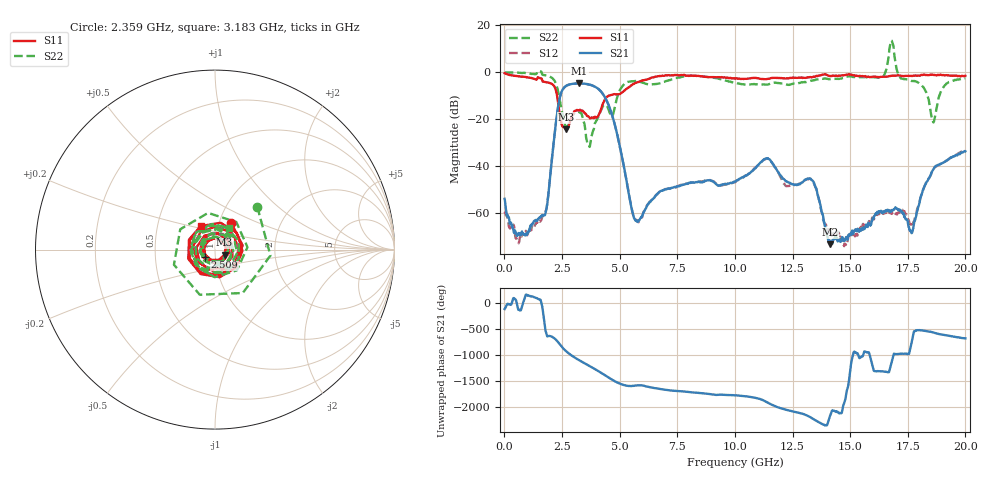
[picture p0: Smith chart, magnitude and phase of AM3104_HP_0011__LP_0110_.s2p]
!Created with skrf (http://scikit-rf.org).
# Hz S RI R 50.0
!freq ReS11 ImS11 ReS21 ImS21 ReS12 ImS12 ReS22 ImS22
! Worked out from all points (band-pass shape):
!   1601 points, 10 MHz to 20 GHz, reference 50 ohm
!   highest |S21| = -4.71 dB at 3.246 GHz (marker M1); lowest = -73.4 dB at 14.13 GHz (marker M2)
!   |S21| within 3 dB of the highest: 2.507 GHz to 4.151 GHz (1.644 GHz wide, 49.4 % of centre)
!   lowest |S11| = -24.3 dB at 2.684 GHz (marker M3), VSWR 1.13, Z = 55.6 - j3.22 ohm
!   |S11| at or under -10 dB: 2.287 GHz to 4.518 GHz (2.232 GHz wide, 65.6 % of centre)
!   |S22| runs from -31.8 to 13.6 dB; largest |S21 - S12| = 0.031
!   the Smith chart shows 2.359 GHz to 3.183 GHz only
!   S11 on the Smith chart (normalised r, x): 2.359 GHz: 1.14, +0.35; 2.509 GHz: 0.89, -0.08; 3.183 GHz: 0.83, +0.23
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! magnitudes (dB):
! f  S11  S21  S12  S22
! 10 MHz  -0.4  -54.0  -59.6  0.0
! 597.2 MHz  -1.7  -69.1  -72.7  -0.1
! 1.734 GHz  -4.0  -61.1  -60.6  -1.2
! 2.359 GHz  -15.2  -13.0  -13.0  -9.5
! 2.509 GHz  -22.9  -7.7  -7.7  -17.7
! 2.684 GHz  -24.3  -5.8  -5.7  -23.1
! 3.183 GHz  -16.2  -4.8  -4.8  -16.8
! 3.246 GHz  -16.3  -4.7  -4.8  -17.0
! 3.346 GHz  -16.3  -4.8  -4.8  -17.7
! 3.658 GHz  -18.9  -5.2  -5.3  -30.6
! 4.533 GHz  -9.9  -14.2  -14.3  -16.2
! 5.695 GHz  -4.5  -63.3  -63.0  -3.7
! 6.682 GHz  -1.6  -51.4  -51.5  -4.8
! 10.01 GHz  -2.7  -46.7  -46.8  -4.5
! 11.4 GHz  -2.8  -36.6  -36.8  -5.2
! 13.34 GHz  -2.1  -45.9  -46.0  -3.6
! 14.13 GHz  -1.6  -73.4  -68.3  -3.0
! 16.36 GHz  -1.9  -59.5  -60.5  -2.3
! 16.68 GHz  -1.6  -59.2  -59.7  7.2
! 17.66 GHz  -1.5  -68.6  -65.3  -3.7
! 18.6 GHz  -1.1  -41.6  -41.8  -21.2
! 20 GHz  -1.5  -33.7  -33.1  -2.5
